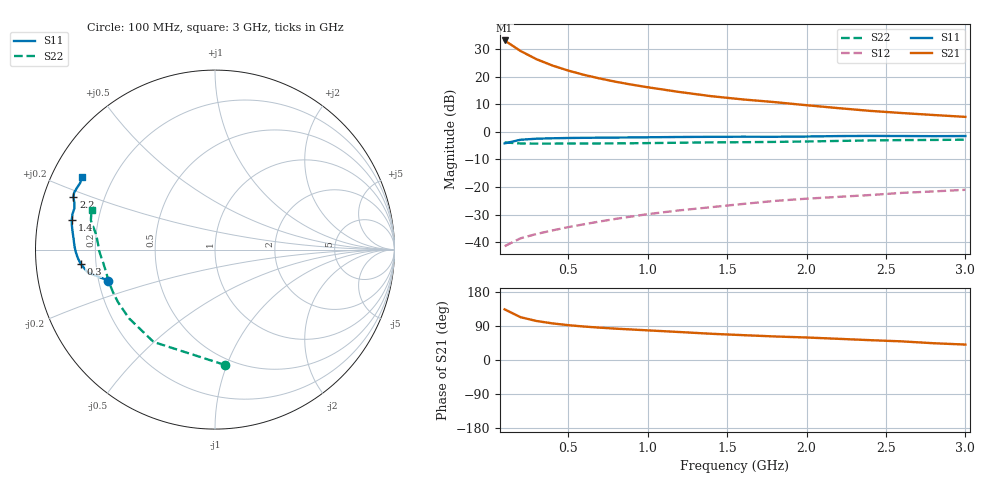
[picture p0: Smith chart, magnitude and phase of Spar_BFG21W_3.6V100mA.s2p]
! Filename: 3_6100bfg21.001
! Title: BFG21W
! Bias: Vce=3.6V; Ic=100mA
! Company: NXP Semiconductors NL
! User: Quality&Reliability T&D
! Measure time: 10 Nov 1999 / 11:44:24
#  MHz  S  MA  R 50
! Freq  S11  S21  S12  S22  :
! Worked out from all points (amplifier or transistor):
!   20 points, 100 MHz to 3 GHz, reference 50 ohm
!   highest |S21| = 33.2 dB at 100 MHz (marker M1)
!   |S21| within 3 dB of that: start of sweep to 178.6 MHz
!   unconditionally stable (mu >= 1): 680.8 MHz to end of sweep
!   at 400 MHz: K = 0.87, MSG = 29.9 dB, |S12| = -35.8 dB
!   at 1.2 GHz: K = 1.06, MAG = 20.0 dB, |S12| = -28.5 dB
!   at 3 GHz: K = 1.05, MAG = 11.9 dB, |S12| = -21.0 dB
!   S11 on the Smith chart (normalised r, x): 100 MHz: 0.24, -0.13; 300 MHz: 0.14, -0.05; 1.4 GHz: 0.10, +0.10; 2.2 GHz: 0.09, +0.18; 3 GHz: 0.09, +0.25
100  0.6186 -163.8  45.7 133.7  0.00845 53.8  0.6444 -85.2
200  0.7205 -169.8  29.45 113.0  0.01173 50.4  0.618 -123.6
300  0.753 -174.0  20.91 103.0  0.01405 53.2  0.6132 -141.4
400  0.7671 -176.8  16.06 96.7  0.0163 56.8  0.6146 -151.3
500  0.7761 -179.1  12.99 92.0  0.01871 59.8  0.6161 -157.6
600  0.7819 179.0  10.85 88.3  0.02112 62.4  0.6172 -162.1
700  0.7859 177.3  9.315 85.3  0.02373 64.5  0.6181 -165.5
800  0.7898 175.8  8.131 82.7  0.02645 66.4  0.6198 -168.4
900  0.7946 174.2  7.209 80.5  0.02922 68.1  0.6229 -170.9
1000  0.7999 172.8  6.471 78.2  0.03218 69.1  0.6269 -173.1
1200  0.8093 170.2  5.308 73.8  0.03772 70.4  0.6369 -176.7
1400  0.8152 168.2  4.454 69.2  0.04309 71.0  0.646 -179.6
1600  0.8183 166.0  3.886 65.6  0.04931 71.5  0.6512 177.8
1800  0.8165 163.5  3.473 62.1  0.056 71.7  0.6591 175.1
2000  0.8251 161.7  3.054 59.4  0.06146 72.3  0.671 172.3
2200  0.8412 159.7  2.704 55.9  0.0663 72.1  0.6861 169.9
2400  0.8466 157.9  2.41 52.3  0.07155 71.4  0.701 168.2
2600  0.843 156.2  2.203 49.2  0.0783 70.4  0.7109 166.7
2800  0.8381 153.8  2.029 44.3  0.08325 68.7  0.7155 164.6
3000  0.8427 151.3  1.876 40.7  0.08907 67.8  0.7227 162.1
